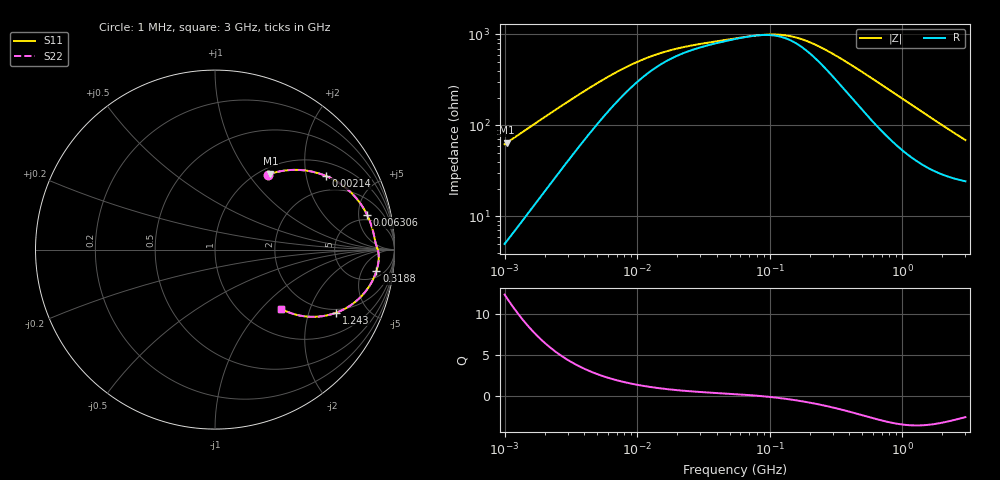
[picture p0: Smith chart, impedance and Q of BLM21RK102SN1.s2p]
! BLM21RK102SN1
# Hz S RI R 50
!Freq.(Hz) S11(Real) S11(Imag) S21(Real) S21(Imag) S12(Real) S12(Imag) S22(Real) S22(Imag)
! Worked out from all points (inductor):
!   401 points, 1 MHz to 3 GHz, reference 50 ohm
!   read as one part in series: L = 9.81 uH near 1.041 MHz
!   highest Q = 12 at 1.041 MHz (marker M1), where L = 9.85 uH
!   self-resonance near 77.79 MHz
!   S11 on the Smith chart (normalised r, x): 1 MHz: 1.10, +1.24; 2.14 MHz: 1.43, +2.60; 6.306 MHz: 4.05, +6.40; 318.8 MHz: 7, -10; 1.243 GHz: 1.84, -3.08; 3 GHz: 1.49, -1.29
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1000000  0.2932 0.4168  0.7068 -0.4168  0.7068 -0.4168  0.2932 0.4168
1040844  0.3091 0.4223  0.6909 -0.4223  0.6909 -0.4223  0.3091 0.4223
1492300  0.4644 0.4441  0.5356 -0.4441  0.5356 -0.4441  0.4644 0.4441
2139570  0.6157 0.4113  0.3843 -0.4113  0.3843 -0.4113  0.6157 0.4113
2831560  0.7099 0.3585  0.2901 -0.3585  0.2901 -0.3585  0.7099 0.3585
3823119  0.7819 0.2926  0.2181 -0.2926  0.2181 -0.2926  0.7819 0.2926
6305767  0.8481 0.1924  0.1519 -0.1924  0.1519 -0.1924  0.8481 0.1924
9794439  0.8735 0.1275  0.1265 -0.1275  0.1265 -0.1275  0.8735 0.1275
1.461624e7  0.8843 0.0863  0.1157 -0.0863  0.1157 -0.0863  0.8843 0.0863
2.41077e7  0.8914 0.0519  0.1086 -0.0519  0.1086 -0.0519  0.8914 0.0519
5.477226e7  0.9014 0.0156  0.0986 -0.0156  0.0986 -0.0156  0.9014 0.0156
8.679508e7  0.9081 -0.0056  0.0919 0.0056  0.0919 0.0056  0.9081 -0.0056
1.171891e8  0.9113 -0.0234  0.0887 0.0234  0.0887 0.0234  0.9113 -0.0234
1.550909e8  0.9124 -0.0438  0.0876 0.0438  0.0876 0.0438  0.9124 -0.0438
2.094008e8  0.9105 -0.0708  0.0895 0.0708  0.0895 0.0708  0.9105 -0.0708
3.188066e8  0.8994 -0.1195  0.1006 0.1195  0.1006 0.1195  0.8994 -0.1195
5.258324e8  0.8634 -0.198  0.1366 0.198  0.1366 0.198  0.8634 -0.198
8.005644e8  0.7972 -0.2777  0.2028 0.2777  0.2028 0.2777  0.7972 -0.2777
1.243477e9  0.6766 -0.3511  0.3234 0.3511  0.3234 0.3511  0.6766 -0.3511
1.54974e9  0.5988 -0.3709  0.4012 0.3709  0.4012 0.3709  0.5988 -0.3709
1.893158e9  0.5237 -0.374  0.4763 0.374  0.4763 0.374  0.5237 -0.374
3e9  0.3666 -0.329  0.6334 0.329  0.6334 0.329  0.3666 -0.329
